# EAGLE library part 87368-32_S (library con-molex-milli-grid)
RECEPTACAL
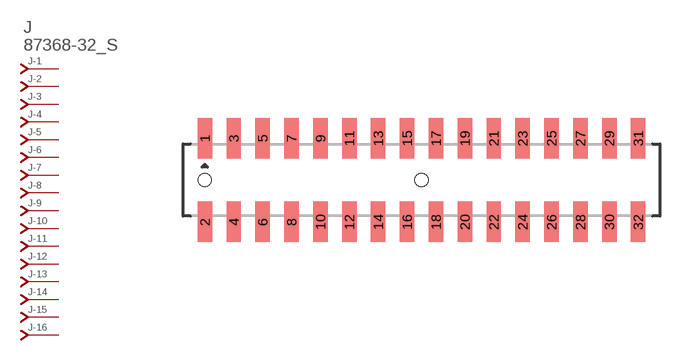
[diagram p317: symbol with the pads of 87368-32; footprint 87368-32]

Designator prefix J; gates -1=J-NV -2=J-N -3=J-N -4=J-N -5=J-N -6=J-N -7=J-N -8=J-N -9=J-N -10=J-N -11=J-N -12=J-N -13=J-N -14=J-N -15=J-N -16=J-N -17=J-N -18=J-N -19=J-N -20=J-N -21=J-N -22=J-N -23=J-N -24=J-N -25=J-N -26=J-N -27=J-N -28=J-N -29=J-N -30=J-N -31=J-N -32=J-N

## 87368-32_S  [87368-32]
1  -1:J  pas
2  -2:J  pas
3  -3:J  pas
4  -4:J  pas
5  -5:J  pas
6  -6:J  pas
7  -7:J  pas
8  -8:J  pas
9  -9:J  pas
10  -10:J  pas
11  -11:J  pas
12  -12:J  pas
13  -13:J  pas
14  -14:J  pas
15  -15:J  pas
16  -16:J  pas
17  -17:J  pas
18  -18:J  pas
19  -19:J  pas
20  -20:J  pas
21  -21:J  pas
22  -22:J  pas
23  -23:J  pas
24  -24:J  pas
25  -25:J  pas
26  -26:J  pas
27  -27:J  pas
28  -28:J  pas
29  -29:J  pas
30  -30:J  pas
31  -31:J  pas
32  -32:J  pas

## Footprint 87368-32 (pad centres in mm)
RECEPTACAL SMD Dual Row, Side Entry
smd 1 x 2.8: 1 -15,2.9; 2 -15,-2.9; 3 -13,2.9; 4 -13,-2.9; 5 -11,2.9; 6 -11,-2.9; 7 -9,2.9; 8 -9,-2.9; 9 -7,2.9; 10 -7,-2.9; 11 -5,2.9; 12 -5,-2.9; 13 -3,2.9; 14 -3,-2.9; 15 -1,2.9; 16 -1,-2.9; 17 1,2.9; 18 1,-2.9; 19 3,2.9; 20 3,-2.9; 21 5,2.9; 22 5,-2.9; 23 7,2.9; 24 7,-2.9; 25 9,2.9; 26 9,-2.9; 27 11,2.9; 28 11,-2.9; 29 13,2.9; 30 13,-2.9; 31 15,2.9; 32 15,-2.9
hole 0.914 at -15,0
hole 0.914 at 0,0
